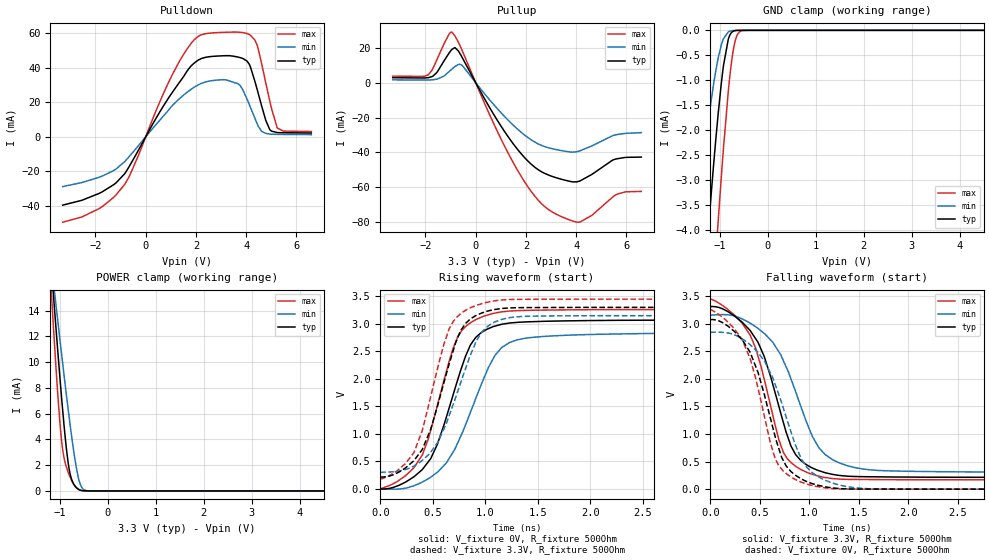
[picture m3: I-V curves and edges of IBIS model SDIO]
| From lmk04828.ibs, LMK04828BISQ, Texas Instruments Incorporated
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|   Model SDIO
[Model]   SDIO
Model_type   I/O
Polarity   Non-Inverting
Enable   Active-Low
Vinl = 0.4
Vinh = 1.6
Vmeas = 1.65
Vref = 3.3
Cref = 0pF
Rref = 500
|   typ   min   max
|   (nom PVT)   (Fast PVT)   (slow PVT)
C_comp   0.555p   0.552p   0.559p
|C_comp (ON state)   0.555p   0.552p   0.559p
|C_comp (OFF state)   0.540p   0.535p   0.544p
| Where   nom PVT is  Nominal Process, 3.3V, 27C
|   Fast PVT is Strong Process, 3.45V, -40C
|   Slow PVT is Weak Process, 3.15V, 125C
[Voltage Range]   3.3   3.15   3.45
[Temperature Range]   27   125   -40
[Pullup Reference]   3.3   3.15   3.45
[Pulldown Reference]   0   0   0
[Power Clamp Reference]   3.3   3.15   3.45
[GND Clamp Reference]   0   0   0
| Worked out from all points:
|   slope of the pulldown table from 0 to 0.495 V, typ, clamps not added: 38.6 ohm
|   slope of the pullup table from 0 to 0.495 V, typ, clamps not added: 38.7 ohm
|   GND clamp passes 1 mA (typ) near -0.96 V on its own axis
|   POWER clamp passes 1 mA (typ) near -0.76 V on its own axis
|   falling waveform, V_fixture 3.3V, R_fixture 500Ohm: 20-80 % time 329ps typ, 396ps min, 304ps max; typ from 3.3 V to 0.213 V
|   rising waveform, V_fixture 0V, R_fixture 500Ohm: 20-80 % time 326ps typ, 386ps min, 298ps max; typ from 0 V to 3.07 V
|   rising waveform, V_fixture 3.3V, R_fixture 500Ohm: 20-80 % time 298ps typ, 337ps min, 281ps max; typ from 0.213 V to 3.3 V
|   falling waveform, V_fixture 0V, R_fixture 500Ohm: 20-80 % time 306ps typ, 352ps min, 293ps max; typ from 3.07 V to 0 V
[Pulldown]
|   Voltage   I(typ)   I(min)   I(max)
-3.3V     -39.51mA   -28.78mA   -49.4mA
-1.855V   -32.74mA   -23.4mA    -41.56mA
-825mV    -21.19mA   -14.19mA   -27.32mA
1.115V    26.94mA    18.95mA    37.59mA
1.808V    41.12mA    27.59mA    54.16mA
2.224V    45.44mA    31.04mA    59.18mA
3.67V     46.25mA    30.83mA    60.66mA
4.165V    40.64mA    17.32mA    58.9mA
4.442V    27.14mA    7.375mA    52.86mA
4.778V    9.588mA    2.062mA    31.25mA
5.234V    2.507mA    1.461mA    5.294mA
6.59V     2.258mA    1.308mA    3.132mA
[GND Clamp]
|   Voltage   I(typ)   I(min)   I(max)
-3.3V     -32.55mA   -22.55mA   -41.85mA
-1.498V   -7.359mA   -3.9mA     -11.04mA
-1.261V   -4.258mA   -1.969mA   -7.206mA
-1.181V   -3.287mA   -1.408mA   -5.977mA
-1.043V   -1.747mA   -592.8uA   -3.933mA
-924mV    -700.9uA   -165.3uA   -2.348mA
-795.3mV  -102.4uA   -18.88uA   -946.5uA
-735.9mV  -26.69uA   -5.763uA   -488.3uA
-676.5mV  -5.707uA   -1.635uA   -195.9uA
-617.1mV  -1.054uA   -434.4nA   -59.58uA
-518.1mV  0A         0A         -5.761uA
6.59V     0A         0A         0A
[Pullup]
|   Voltage   I(typ)   I(min)   I(max)
-3.3V     2.838mA    1.604mA    3.746mA
-1.884V   2.87mA     1.509mA    4.457mA
-1.548V   5.78mA     2.005mA    12.97mA
-943.8mV  19.07mA    7.823mA    28.97mA
-825mV    20.11mA    9.247mA    26.79mA
-537.9mV  14.47mA    9.821mA    18.44mA
1.393V    -33.02mA   -22.93mA   -43.08mA
2.175V    -46.23mA   -32.41mA   -61.62mA
2.779V    -52.18mA   -36.79mA   -71.39mA
4.135V    -56.37mA   -39.1mA    -79.87mA
5.61V     -43.62mA   -29.77mA   -63.95mA
6.59V     -42.62mA   -28.62mA   -62.29mA
[POWER Clamp]
|   Voltage   I(typ)   I(min)   I(max)
-3.3V     125mA      90.16mA    153.8mA
-1.181V   17.55mA    17.82mA    15.64mA
-1.171V   17.06mA    17.48mA    15.02mA
-1.132V   15.11mA    16.15mA    12.59mA
-1.082V   12.71mA    14.5mA     9.663mA
-1.003V   8.987mA    11.89mA    5.49mA
-943.8mV  6.36mA     9.97mA     3.265mA
-854.7mV  2.98mA     7.172mA    1.743mA
-795.3mV  1.474mA    5.393mA    1.144mA
-587.4mV  82.22uA    656.7uA    72.92uA
-399.3mV  793.6nA    8.386uA    949.6nA
6.59V     0A         0A         0A
[Ramp]
R_load = 500
|   typ   min   max
dV/dt_r   1.84196/3.25658e-10   1.70003/3.86019e-10   1.95703/2.97502e-10
dV/dt_f   1.85143/3.29443e-10   1.70554/3.95766e-10   1.96811/3.03724e-10
[Falling Waveform]
V_fixture = 3.3V
V_fixture_min = 3.15V
V_fixture_max = 3.45V
R_fixture = 500Ohm
C_fixture = 0F
|   Time   V(typ)   V(min)   V(max)
|   0   3.29918   3.14939   3.4489
|   3.05961e-10   3.29974   3.15076   3.45063
|   3.33339e-10   3.2998   3.15088   3.44867
|   3.49696e-10   3.29983   3.15096   3.45073
|   3.7197e-10   3.29987   3.15106   3.45767
|   3.81982e-10   3.30076   3.1511   3.46079
|   3.9416e-10   3.30184   3.15116   3.46138
|   4.21359e-10   3.30778   3.15128   3.46269
|   4.37665e-10   3.31134   3.15135   3.46262
|   4.40642e-10   3.31199   3.15136   3.4624
|   4.5457e-10   3.31257   3.15143   3.46139
|   4.57469e-10   3.31269   3.15181   3.46118
|   4.81152e-10   3.31367   3.15493   3.4548
|   4.96532e-10   3.31431   3.15696   3.44636
|   5.09584e-10   3.31388   3.15868   3.4392
|   5.18674e-10   3.31358   3.15988   3.43148
|   5.44583e-10   3.30921   3.1633   3.40948
|   5.46033e-10   3.30897   3.16349   3.40792
|   5.48352e-10   3.30801   3.16379   3.40542
|   5.78563e-10   3.29551   3.16532   3.37289
|   5.90087e-10   3.28753   3.16591   3.36048
|   6.03354e-10   3.27834   3.16658   3.34357
|   6.1802e-10   3.26819   3.16663   3.32488
|   6.28911e-10   3.25785   3.16668   3.311
|   6.51977e-10   3.23595   3.16528   3.2816
|   6.61126e-10   3.22727   3.16473   3.26774
|   6.66968e-10   3.22172   3.16342   3.25888
|   7.00803e-10   3.1819   3.15583   3.2076
|   7.31147e-10   3.14618   3.14217   3.1616
|   7.31977e-10   3.14498   3.1418   3.16035
|   7.49024e-10   3.12021   3.13412   3.12814
|   8.07064e-10   3.0359   3.09325   3.01849
|   8.11147e-10   3.02997   3.08945   3.01078
|   8.11977e-10   3.02843   3.08868   3.00921
|   8.79822e-10   2.90206   3.02562   2.82758
|   8.91147e-10   2.88097   3.01248   2.79727
|   8.91977e-10   2.87874   3.01152   2.79504
|   9.48139e-10   2.72804   2.94639   2.55692
|   9.59822e-10   2.6967   2.93284   2.48499
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0s        3.299V     3.149V     3.449V
322.7ps   3.028V     3.089V     3.009V
481.9ps   2.666V     2.917V     2.415V
610.7ps   2.034V     2.704V     1.499V
738.9ps   1.204V     2.327V     664.1mV
814.9ps   781.7mV    1.999V     484.4mV
917.3ps   517.3mV    1.486V     353.4mV
1.096ns   336.4mV    753.8mV    236.8mV
1.381ns   237mV      427.5mV    178mV
3.511ns   213.5mV    306.8mV    168.7mV
[Rising Waveform]
V_fixture = 0V
V_fixture_min = 0V
V_fixture_max = 0V
R_fixture = 500Ohm
C_fixture = 0F
|   Time   V(typ)   V(min)   V(max)
|   0   0.000216606   0.000221736   0.000222674
|   3.05961e-10   0.00188786   0.00166472   0.00210063
|   3.14751e-10   0.00193588   0.00170618   0.00115131
|   3.30086e-10   0.00201964   0.0017785   -0.00222556
|   3.48683e-10   0.00165817   0.00186621   -0.00632068
|   3.49696e-10   0.00151214   0.00187099   -0.00654379
|   3.55943e-10   0.000611772   0.00190045   -0.0066957
|   3.749e-10   -0.0021205   0.00198986   -0.00445632
|   4.0401e-10   -0.0063161   0.00212715   -0.0056536
|   4.20415e-10   -0.00661064   0.00220452   -0.00632835
|   4.37665e-10   -0.00692034   0.000207302   -0.00703785
|   4.57469e-10   -0.00727589   -0.00208553   -0.0066641
|   4.81152e-10   -0.00770108   -0.00482749   -0.00322723
|   4.89304e-10   -0.00784744   -0.00577137   -0.000298967
|   5.09584e-10   -0.00821153   -0.00648651   0.00698524
|   5.18674e-10   -0.00837473   -0.00680706   0.0134294
|   5.46033e-10   -0.00577592   -0.00777184   0.0328247
|   5.78563e-10   0.00322819   -0.00891898   0.055886
|   5.90087e-10   0.0088856   -0.00932534   0.0640553
|   6.1802e-10   0.0225995   -0.0103104   0.0927645
|   6.28911e-10   0.0302428   -0.0106944   0.103957
|   6.51977e-10   0.0464318   -0.00980895   0.127664
|   6.61126e-10   0.0528532   -0.00945773   0.139846
|   6.66968e-10   0.0569531   -0.00848675   0.147624
|   7.00803e-10   0.088319   -0.00286288   0.192673
|   7.31147e-10   0.11645   0.00798168   0.233076
|   7.31977e-10   0.117458   0.00827813   0.23418
|   7.49024e-10   0.13818   0.0143705   0.264953
|   8.07064e-10   0.208729   0.0474054   0.369722
|   8.11147e-10   0.213692   0.0506691   0.377092
|   8.11977e-10   0.215051   0.0513322   0.378589
|   8.79822e-10   0.326246   0.105564   0.577039
|   8.91147e-10   0.344808   0.117637   0.610167
|   8.91977e-10   0.346868   0.118521   0.612593
|   9.48139e-10   0.486329   0.178384   0.899114
|   9.59822e-10   0.515339   0.190837   0.979767
|   9.71147e-10   0.543463   0.206941   1.05795
|   1.00524e-09   0.682049   0.25542   1.29333
|   1.03413e-09   0.799463   0.296492   1.50624
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0s        216.6uV    221.7uV    222.7uV
320.7ps   215.1mV    51.33mV    378.6mV
400.7ps   346.9mV    118.5mV    612.6mV
479.9ps   543.5mV    206.9mV    1.058V
736.9ps   1.975V     828.2mV    2.758V
812.9ps   2.413V     1.164V     2.948V
915.3ps   2.762V     1.667V     3.08V
1.094ns   2.957V     2.427V     3.194V
1.303ns   3.024V     2.706V     3.238V
3.509ns   3.07V      2.834V     3.262V
[Rising Waveform]
V_fixture = 3.3V
V_fixture_min = 3.15V
V_fixture_max = 3.45V
R_fixture = 500Ohm
C_fixture = 0F
|   Time   V(typ)   V(min)   V(max)
|   0   0.212627   0.303576   0.16845
|   2.24e-10   0.212833   0.304017   0.168721
|   2.7382e-10   0.213493   0.303838   0.169609
|   3.05961e-10   0.213919   0.304254   0.170182
|   3.14751e-10   0.214036   0.304368   0.169211
|   3.30086e-10   0.214239   0.304566   0.16544
|   3.40881e-10   0.21399   0.304706   0.162786
|   3.48683e-10   0.21381   0.304807   0.162163
|   3.55943e-10   0.212837   0.304901   0.161583
|   3.61665e-10   0.21207   0.304975   0.162363
|   3.68484e-10   0.211156   0.305063   0.163442
|   3.749e-10   0.210296   0.305146   0.163941
|   3.81982e-10   0.209347   0.305237   0.163891
|   3.95702e-10   0.207508   0.305415   0.163594
|   4.0401e-10   0.206395   0.305274   0.163414
|   4.11747e-10   0.20661   0.305142   0.163246
|   4.20415e-10   0.206874   0.304994   0.163058
|   4.21359e-10   0.206903   0.304895   0.163038
|   4.37886e-10   0.207407   0.303161   0.163622
|   4.57469e-10   0.208004   0.30103   0.164315
|   4.74256e-10   0.208516   0.299203   0.16749
|   4.81152e-10   0.208726   0.298909   0.168794
|   4.96532e-10   0.209195   0.298253   0.175443
|   5.0415e-10   0.209745   0.297928   0.178736
|   5.09584e-10   0.210136   0.298185   0.181085
|   5.16037e-10   0.210602   0.29849   0.185542
|   5.18674e-10   0.210792   0.298665   0.187364
|   5.44583e-10   0.215429   0.300382   0.20526
|   5.46033e-10   0.215689   0.300478   0.206624
|   5.78563e-10   0.228236   0.302635   0.237236
|   5.90087e-10   0.235631   0.303399   0.24808
|   6.03354e-10   0.244145   0.304278   0.264343
|   6.1802e-10   0.253557   0.306029   0.282321
|   6.28911e-10   0.263341   0.307329   0.29567
|   6.51977e-10   0.284066   0.311731   0.323944
|   6.61126e-10   0.292286   0.313477   0.339065
|   6.66968e-10   0.297535   0.31624   0.348719
|   7.31147e-10   0.374616   0.346603   0.454788
|   7.31977e-10   0.375985   0.346996   0.456159
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0s        212.6mV    303.6mV    168.4mV
320.7ps   508.8mV    411mV      655.2mV
400.7ps   713.5mV    513.6mV    1.058V
468.5ps   1.025V     629.6mV    1.579V
653.4ps   2.25V      1.312V     2.895V
764.3ps   2.87V      1.917V     3.18V
863ps     3.093V     2.448V     3.294V
1.03ns    3.233V     2.964V     3.395V
1.232ns   3.287V     3.111V     3.44V
3.509ns   3.299V     3.149V     3.449V
[Falling Waveform]
|Gnd
V_fixture = 0V
V_fixture_min = 0V
V_fixture_max = 0V
R_fixture = 500Ohm
C_fixture = 0F
|   Time   V(typ)   V(min)   V(max)
|   0   3.07227   2.83991   3.26292
|   2.24e-10   3.07251   2.84035   3.2632
|   2.34428e-10   3.07254   2.84036   3.26338
|   3.05961e-10   3.07342   2.84043   3.26462
|   3.33339e-10   3.07376   2.84046   3.26268
|   3.48683e-10   3.07394   2.84048   3.26449
|   3.49696e-10   3.0739   2.84048   3.26461
|   3.50283e-10   3.07388   2.84048   3.2648
|   3.7197e-10   3.07297   2.84078   3.27184
|   3.749e-10   3.0732   2.84082   3.27279
|   3.9416e-10   3.07467   2.84109   3.27404
|   3.98131e-10   3.07545   2.84114   3.2743
|   4.0839e-10   3.07746   2.84128   3.27411
|   4.21359e-10   3.08001   2.84147   3.27356
|   4.3112e-10   3.08192   2.8416   3.27289
|   4.37665e-10   3.08226   2.84169   3.27244
|   4.51451e-10   3.08295   2.84188   3.27053
|   4.5457e-10   3.08287   2.84193   3.2701
|   4.57469e-10   3.0828   2.84216   3.26969
|   4.64182e-10   3.08263   2.84269   3.26742
|   4.81152e-10   3.08094   2.84405   3.26166
|   5.09584e-10   3.07811   2.84632   3.24292
|   5.18674e-10   3.07721   2.84704   3.23397
|   5.44583e-10   3.06999   2.84911   3.20845
|   5.46033e-10   3.06959   2.84923   3.20665
|   5.48352e-10   3.06831   2.84941   3.20377
|   5.64515e-10   3.05937   2.84904   3.18371
|   5.78563e-10   3.05161   2.84792   3.16627
|   5.90087e-10   3.04149   2.84699   3.15197
|   6.03354e-10   3.02985   2.84593   3.13222
|   6.1802e-10   3.01698   2.84401   3.11038
|   6.28911e-10   3.00418   2.84258   3.09416
|   6.51977e-10   2.97706   2.83784   3.05982
|   6.61126e-10   2.96631   2.83596   3.04297
|   6.66968e-10   2.95944   2.83371   3.03221
|   7.00803e-10   2.90945   2.82067   2.96991
|   7.31147e-10   2.86461   2.80058   2.91403
|   7.31977e-10   2.86302   2.80003   2.9125
|   7.49024e-10   2.83029   2.78874   2.86919
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0s        3.072V     2.84V      3.263V
128.7ps   3.017V     2.844V     3.11V
322.7ps   2.709V     2.726V     2.709V
470.5ps   2.172V     2.505V     1.918V
655.5ps   950.5mV    1.899V     551.8mV
766.3ps   420.8mV    1.309V     284.7mV
865ps     247.1mV    779.5mV    170.5mV
1.032ns   99.93mV    295.9mV    65.69mV
1.381ns   5.268mV    46.54mV    2.417mV
3.511ns   321.9uV    459.9uV    306.4uV
